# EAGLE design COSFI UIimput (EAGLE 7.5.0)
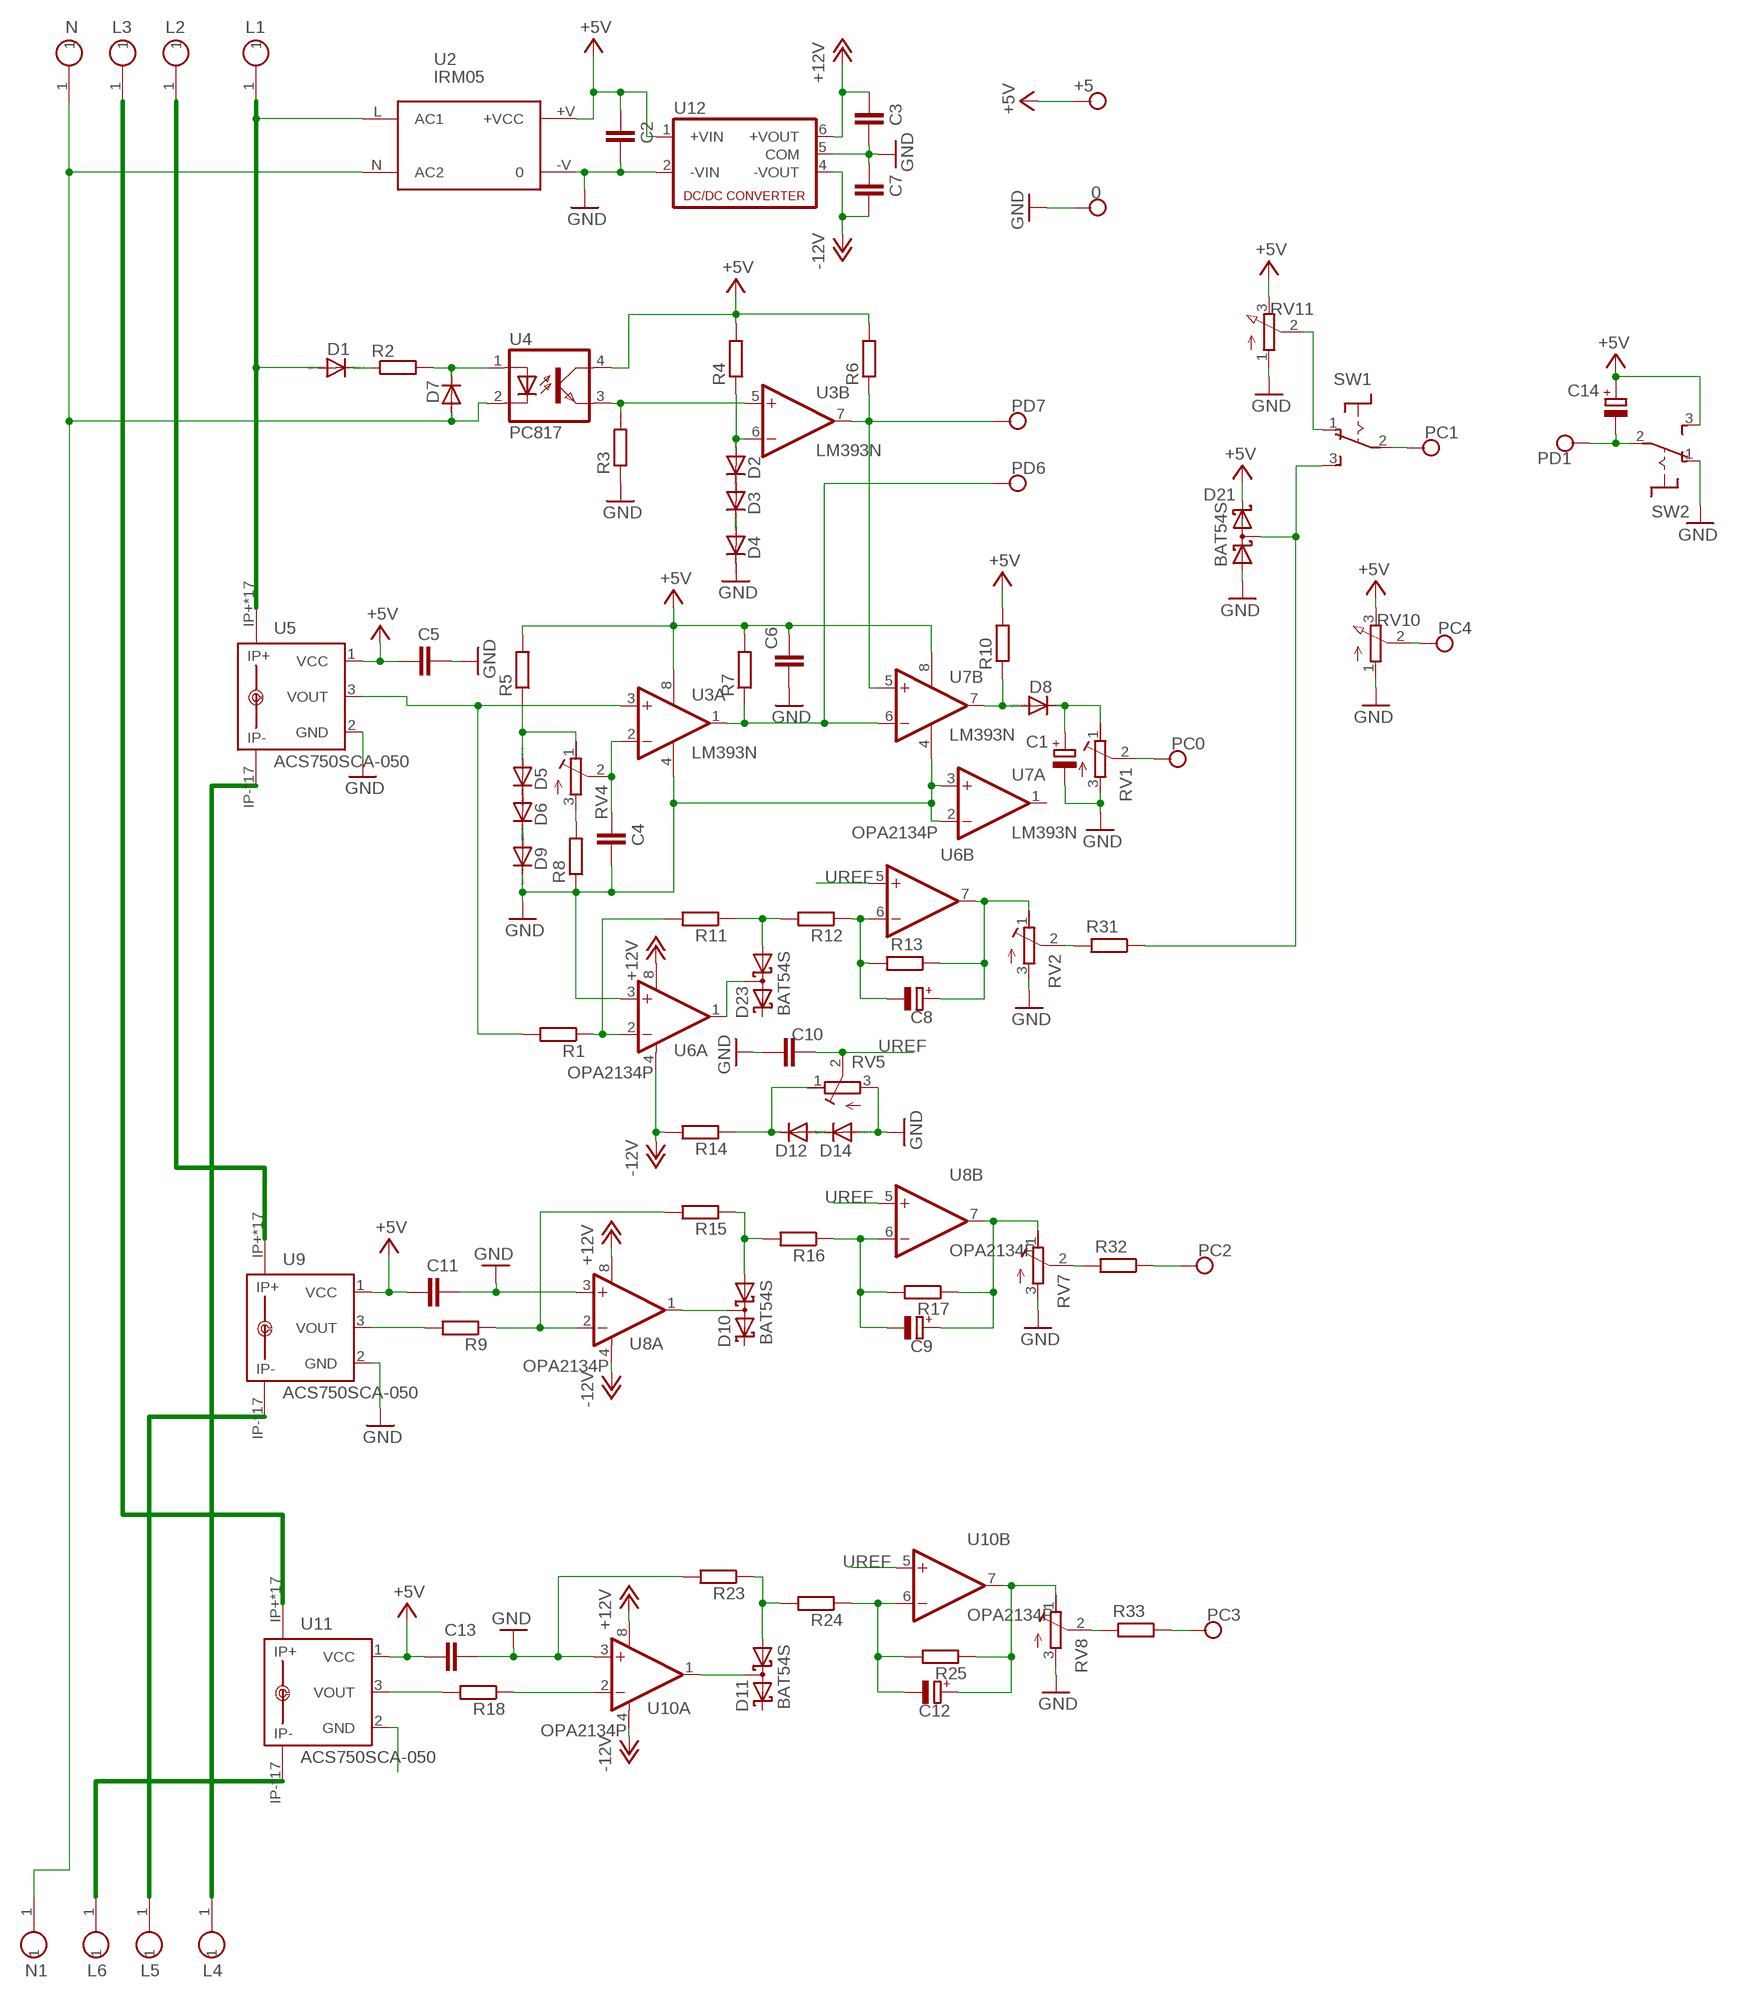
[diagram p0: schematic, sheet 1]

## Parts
0  CONNWIRE  [CONNWIRE]
+5  CONNWIRE  [CONNWIRE]
C1  CPOL-EUE2-5  [E2-5]
C2  C-EUC1206  [C1206]
C3  C-EUC1206  [C1206]
C4  C-EUC1206  [C1206]
C5  C-EUC1206  [C1206]
C6  C-EUC1206  [C1206]
C7  C-EUC1206  [C1206]
C8  CPOL-EUE2-5  [E2-5]
C9  CPOL-EUE2-5  [E2-5]
C10  C-EUC1206  [C1206]
C11  C-EUC1206  [C1206]
C12  CPOL-EUE2-5  [E2-5]
C13  C-EUC1206  [C1206]
C14  CPOL-EUE2-5  [E2-5]
D1  1N4004  [DO41-10]
D2  1N4148DO35-7  [DO35-7]
D3  1N4148DO35-7  [DO35-7]
D4  1N4148DO35-7  [DO35-7]
D5  1N4148DO35-7  [DO35-7]
D6  1N4148DO35-7  [DO35-7]
D7  1N4004  [DO41-10]
D8  1N4148DO35-7  [DO35-7]
D9  1N4148DO35-7  [DO35-7]
D10  BAT54S  [SOT23]
D11  BAT54S  [SOT23]
D12  1N4148DO35-7  [DO35-7]
D14  1N4148DO35-7  [DO35-7]
D21  BAT54S  [SOT23]
D23  BAT54S  [SOT23]
L1  CONNHOLE  [CONNHOLE4]
L2  CONNHOLE  [CONNHOLE4]
L3  CONNHOLE  [CONNHOLE4]
L4  CONNHOLE  [CONNHOLE4]
L5  CONNHOLE  [CONNHOLE4]
L6  CONNHOLE  [CONNHOLE4]
N  CONNHOLE  [CONNHOLE4]
N1  CONNHOLE  [CONNHOLE4]
PC0  CONNWIRE  [CONNWIRE]
PC1  CONNWIRE  [CONNWIRE]
PC2  CONNWIRE  [CONNWIRE]
PC3  CONNWIRE  [CONNWIRE]
PC4  CONNWIRE  [CONNWIRE]
PD1  CONNWIRE  [CONNWIRE]
PD6  CONNWIRE  [CONNWIRE]
PD7  CONNWIRE  [CONNWIRE]
R1  R-EU_0204/7  [0204/7]
R2  R-EU_0617/22  [0617/22]
R3  R-EU_0204/7  [0204/7]
R4  R-EU_0204/7  [0204/7]
R5  R-EU_0204/7  [0204/7]
R6  R-EU_0204/7  [0204/7]
R7  R-EU_0204/7  [0204/7]
R8  R-EU_0204/7  [0204/7]
R9  R-EU_0204/7  [0204/7]
R10  R-EU_0204/7  [0204/7]
R11  R-EU_0204/7  [0204/7]
R12  R-EU_0204/7  [0204/7]
R13  R-EU_0204/7  [0204/7]
R14  R-EU_0204/7  [0204/7]
R15  R-EU_0204/7  [0204/7]
R16  R-EU_0204/7  [0204/7]
R17  R-EU_0204/7  [0204/7]
R18  R-EU_0204/7  [0204/7]
R23  R-EU_0204/7  [0204/7]
R24  R-EU_0204/7  [0204/7]
R25  R-EU_0204/7  [0204/7]
R31  R-EU_0204/7  [0204/7]
R32  R-EU_0204/7  [0204/7]
R33  R-EU_0204/7  [0204/7]
RV1  R-TRIMM-3386-F  [R-TRIMM-3386F]
RV2  R-TRIMM-3386-F  [R-TRIMM-3386F]
RV4  R-TRIMM-3386-F  [R-TRIMM-3386F]
RV5  R-TRIMM-3386-F  [R-TRIMM-3386F]
RV7  R-TRIMM-3386-F  [R-TRIMM-3386F]
RV8  R-TRIMM-3386-F  [R-TRIMM-3386F]
RV10  PTV09A  PV09A  [PTV09]
RV11  PTV09A  PV09A  [PTV09]
SW1  8MS9P1  [8MS9]
SW2  8MS9P1  [8MS9]
U2  IRM05  [IRM05]
U3  LM393N  [DIL08]
U4  PC817  [DIL04]
U5  ACS750SCA-050  [ACS75050]
U6  OPA2134P  [DIL08]
U7  LM393N  [DIL08]
U8  OPA2134P  [DIL08]
U9  ACS750SCA-050  [ACS75050]
U10  OPA2134P  [DIL08]
U11  ACS750SCA-050  [ACS75050]
U12  NMA  [NMA]

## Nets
+5V: +5.P$1 C2.1 C5.2 C6.2 C11.2 C13.2 C14.+ D21.2(C2) R4.2 R5.2 R6.2 R7.2 R10.2 RV10.3(E) RV11.3(E) SW2.3(S) U2.+V(+VCC) U3.8(P:V+) U4.4(COL) U5.1(VCC) U7.8(P:V+) U9.1(VCC) U11.1(VCC) U12.1(+VIN)
+12V: C3.1 U6.8(A:V+) U8.8(A:V+) U10.8(A:V+) U12.6(+VOUT)
-12V: C7.2 R14.2 U6.4(A:V-) U8.4(A:V-) U10.4(A:V-) U12.4(-VOUT)
GND: 0.P$1 C1.- C2.2 C3.2 C4.2 C5.1 C6.1 C7.1 C10.1 C11.1 C13.1 D4.C D9.C D14.A D21.1(A1) R3.1 R8.1 R23.2 RV1.3(E) RV2.3(E) RV5.3(E) RV7.3(E) RV8.3(E) RV10.1(A) RV11.1(A) SW2.1(O) U2.-V U3.4(P:V-) U5.2(GND) U6.3(A:+IN) U7.2(A:-IN) U7.3(A:+IN) U7.4(P:V-) U8.3(A:+IN) U9.2(GND) U10.3(A:+IN) U11.2(GND) U12.2(-VIN) U12.5(COM)
N$1: D1.C R2.1
N$2: R1.1 R11.2 U6.2(A:-IN)
N$3: D7.C R2.2 U4.1(A)
N$4: D2.C D3.A
N$5: D7.A N1.1 N.1 U2.N(AC2) U4.2(C)
N$6: D1.A L1.1 U2.L(AC1) U5.IP+ U5.IP+@2(IP+) U5.IP+@3(IP+) U5.IP+@4(IP+) U5.IP+@5(IP+) U5.IP+@6(IP+) U5.IP+@7(IP+) U5.IP+@8(IP+) U5.IP+@9(IP+) U5.IP+@10(IP+) U5.IP+@11(IP+) U5.IP+@12(IP+) U5.IP+@13(IP+) U5.IP+@14(IP+) U5.IP+@15(IP+) U5.IP+@16(IP+) U5.IP+@17(IP+)
N$7: RV11.2(S) SW1.1(O)
N$8: D3.C D4.A
N$9: D12.A D14.C
N$10: D12.C R14.1 RV5.1(A)
N$11: R8.2 RV4.3(E)
N$12: D5.A R5.1 RV4.1(A)
N$13: R3.2 U3.5(B:+IN) U4.3(EMIT)
N$14: R1.2 U3.3(A:+IN) U5.3(VOUT)
N$15: D5.C D6.A
N$16: D2.A R4.1 U3.6(B:-IN)
N$17: D8.A R10.1 U7.7(B:OUT)
N$18: PD7.P$1 R6.1 U3.7(B:OUT) U7.5(B:+IN)
N$19: D6.C D9.A
N$20: PD6.P$1 R7.1 U3.1(A:OUT) U7.6(B:-IN)
N$21: C4.1 RV4.2(S) U3.2(A:-IN)
N$22: C1.+ D8.C RV1.1(A)
N$23: PC0.P$1 RV1.2(S)
N$24: D23.3(C1A2) U6.1(A:OUT)
N$25: PC1.P$1 SW1.2(P)
N$26: PC4.P$1 RV10.2(S)
N$27: D21.3(C1A2) R31.1 SW1.3(S)
N$28: C14.- PD1.P$1 SW2.2(P)
N$29: R9.1 R15.2 U8.2(A:-IN)
N$31: D23.1(A1) R11.1 R12.2
N$32: C8.- R12.1 R13.2 U6.6(B:-IN)
N$33: C8.+ R13.1 RV2.1(A) U6.7(B:OUT)
N$35: R31.2 RV2.2(S)
N$36: L2.1 U9.IP+ U9.IP+@2(IP+) U9.IP+@3(IP+) U9.IP+@4(IP+) U9.IP+@5(IP+) U9.IP+@6(IP+) U9.IP+@7(IP+) U9.IP+@8(IP+) U9.IP+@9(IP+) U9.IP+@10(IP+) U9.IP+@11(IP+) U9.IP+@12(IP+) U9.IP+@13(IP+) U9.IP+@14(IP+) U9.IP+@15(IP+) U9.IP+@16(IP+) U9.IP+@17(IP+)
N$37: D10.3(C1A2) U8.1(A:OUT)
N$39: R9.2 U9.3(VOUT)
N$40: D10.1(A1) R15.1 R16.2
N$41: C9.- R16.1 R17.2 U8.6(B:-IN)
N$42: C9.+ R17.1 RV7.1(A) U8.7(B:OUT)
N$43: PC2.P$1 R32.1
N$44: L3.1 U11.IP+ U11.IP+@2(IP+) U11.IP+@3(IP+) U11.IP+@4(IP+) U11.IP+@5(IP+) U11.IP+@6(IP+) U11.IP+@7(IP+) U11.IP+@8(IP+) U11.IP+@9(IP+) U11.IP+@10(IP+) U11.IP+@11(IP+) U11.IP+@12(IP+) U11.IP+@13(IP+) U11.IP+@14(IP+) U11.IP+@15(IP+) U11.IP+@16(IP+) U11.IP+@17(IP+)
N$45: R32.2 RV7.2(S)
N$46: R18.1 U10.2(A:-IN)
N$47: R18.2 U11.3(VOUT)
N$48: D11.3(C1A2) U10.1(A:OUT)
N$49: D11.1(A1) R23.1 R24.2
N$50: C12.- R24.1 R25.2 U10.6(B:-IN)
N$51: C12.+ R25.1 RV8.1(A) U10.7(B:OUT)
N$52: PC3.P$1 R33.1
N$53: R33.2 RV8.2(S)
N$54: L4.1 U5.IP- U5.IP-@2(IP-) U5.IP-@3(IP-) U5.IP-@4(IP-) U5.IP-@5(IP-) U5.IP-@6(IP-) U5.IP-@7(IP-) U5.IP-@8(IP-) U5.IP-@9(IP-) U5.IP-@10(IP-) U5.IP-@11(IP-) U5.IP-@12(IP-) U5.IP-@13(IP-) U5.IP-@14(IP-) U5.IP-@15(IP-) U5.IP-@16(IP-) U5.IP-@17(IP-)
N$55: L5.1 U9.IP- U9.IP-@2(IP-) U9.IP-@3(IP-) U9.IP-@4(IP-) U9.IP-@5(IP-) U9.IP-@6(IP-) U9.IP-@7(IP-) U9.IP-@8(IP-) U9.IP-@9(IP-) U9.IP-@10(IP-) U9.IP-@11(IP-) U9.IP-@12(IP-) U9.IP-@13(IP-) U9.IP-@14(IP-) U9.IP-@15(IP-) U9.IP-@16(IP-) U9.IP-@17(IP-)
N$57: L6.1 U11.IP- U11.IP-@2(IP-) U11.IP-@3(IP-) U11.IP-@4(IP-) U11.IP-@5(IP-) U11.IP-@6(IP-) U11.IP-@7(IP-) U11.IP-@8(IP-) U11.IP-@9(IP-) U11.IP-@10(IP-) U11.IP-@11(IP-) U11.IP-@12(IP-) U11.IP-@13(IP-) U11.IP-@14(IP-) U11.IP-@15(IP-) U11.IP-@16(IP-) U11.IP-@17(IP-)
UREF: C10.2 RV5.2(S) U6.5(B:+IN) U8.5(B:+IN) U10.5(B:+IN)
Unconnected: D10.2(C2) D11.2(C2) D23.2(C2) U7.1(A:OUT)

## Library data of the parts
0 +5 PC0 PC1-PC4 PD1 PD6 PD7 = connholes:CONNWIRE
C1 C8 C9 C12 C14 = rcl:CPOL-EU: POLARIZED CAPACITOR, European symbol
C2-C7 C10 C11 C13 = rcl:C-EU: CAPACITOR, European symbol
D1 D7 = diode:1N4004: DIODE
D2-D6 D8 D9 D12 D14 = diode:1N4148: DIODE
D10 D11 D21 D23 = diode:BAT54S: Schottky Diodes Pin connection corrected 2011-05-04 Source: Fairchild .. BAT54.pdf
L1-L6 N N1 = connholes:CONNHOLE
R1-R18 R23-R25 R31-R33 = rcl:R-EU_: RESISTOR, European symbol
RV1 RV2 RV4 RV5 RV7 RV8 = rcl:R-TRIMM-3386-F
RV10 RV11 = pot:PV09A
SW1 SW2 = switch:8MS9P1
U2 = acdc:IRM05: ACDC connector
U3 U7 = linear:LM393: COMPARATOR
U4 = optocoupler:PC817: SHARP OPTO COUPLER; MPN: PC817X4J000F; OC_FARNELL: 9707727; OC_NEWARK: 97K7059
U5 U9 U11 = allegro:ACS750*CA-050: Current Sensor display layer 49 Reference in BRD and place VIAs on circles Source: www.allegromicro.com/datafile/0750-050.pdf; MF: ALLEGRO MICROSYSTEMS, INC.; MPN: ACS750SCA-050; OC_FARNELL: 1457175; OC_NEWARK: 81H6588
U6 U8 U10 = burr-brown:OPA2134: Operational Amplifier; MF: TEXAS INSTRUMENTS; MPN: OPA2134PA; OC_FARNELL: 1097574; OC_NEWARK: 74K3897
U12 = dc-dc-converter:NMA: DC-DC CONVERTER; MF: C & D TECHNOLOGIES, INC; MPN: NMA0515SC; OC_FARNELL: 1021434; OC_NEWARK: 61K3064

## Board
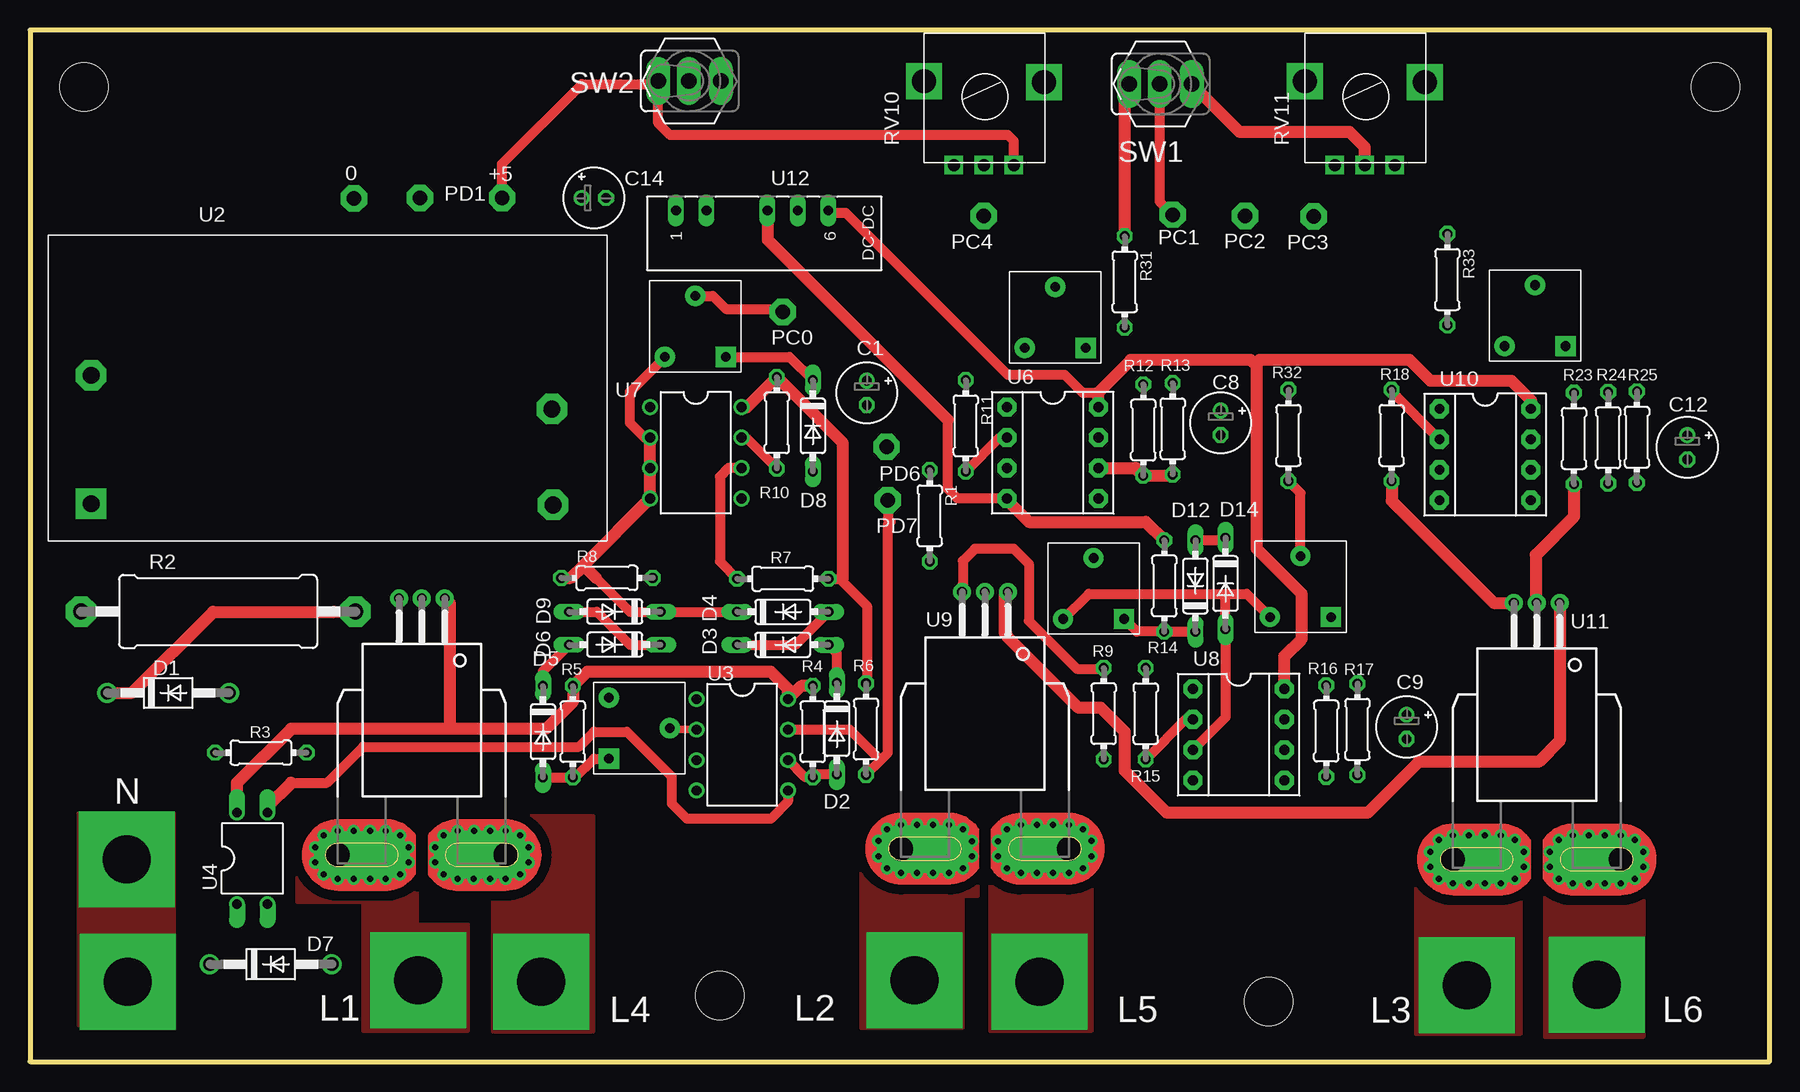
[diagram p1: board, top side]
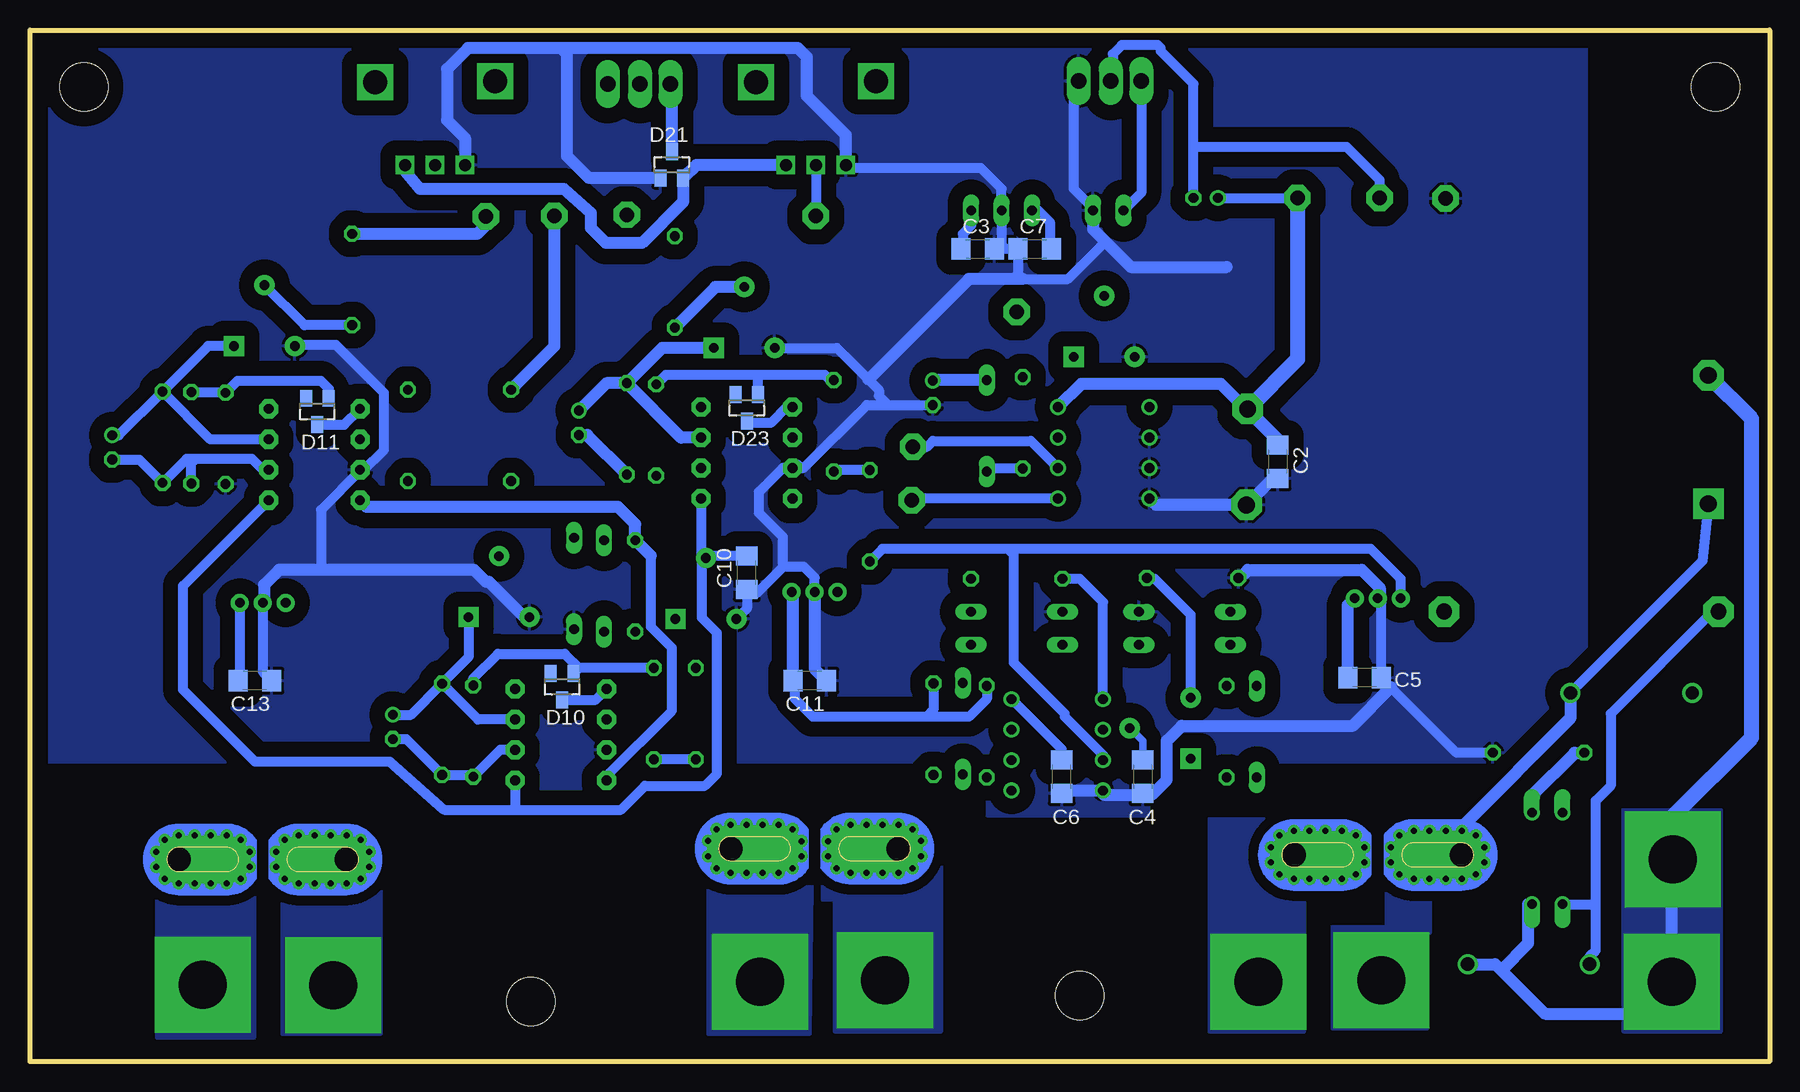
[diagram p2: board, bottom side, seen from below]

Size 145 x 86 mm. Coordinates in mm from the lower left corner, seen from the top.
Outline: 0,0 145,0 145,86 0,86 0,0
Copper layers (1*16): Top 0.035mm / dielectric 1.5mm / Bottom 0.035mm
Design rules "default": minimum track width 10mil, minimum drill 24mil, track to track 8mil, track to pad 8mil, pad to pad 8mil, via to via 8mil, smd to smd 8mil, copper to edge 40mil, drill to drill 8mil, minimum pad ring 10mil, minimum via ring 8mil, stop-mask expansion 4mil, vias tented up to drill 0mil, thermal gap 10mil
Holes 4 mm at 57.5,5.5 103.25,5 140.5,81.25 4.5,81.25
bRestrict: area 57.9,32.4 to 67.1,41.6

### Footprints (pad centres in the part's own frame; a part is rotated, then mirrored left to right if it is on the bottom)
CONNWIRE = drill 1.2 pad 2.184 octagon: P$1 0,0
E2-5 = drill 0.813 pad 1.27: + -1.016,0 | drill 0.813 pad 1.27 octagon: - 1.016,0
C1206 = smd 1.6 x 1.8: 1 -1.4,0; 2 1.4,0
DO41-10 = drill 1.118: A 5.08,0; C -5.08,0
DO35-7 = drill 0.813 long: A 3.81,0; C -3.81,0
SOT23 = smd 1 x 1.4: 1 -0.95,-1.1; 2 0.95,-1.1; 3 0,1.1
CONNHOLE4 = drill 4 pad 8 square: 1 0,0
0204/7 = drill 0.813 octagon: 1 -3.81,0; 2 3.81,0
0617/22 = drill 1.3 pad 2.54 octagon: 1 -11.43,0; 2 11.43,0
R-TRIMM-3386F = drill 0.8 pad 1.676 square: 1 0,0 | drill 0.8 pad 1.676: 2 5.08,2.54; 3 0,5.08
PTV09 = drill 1 square: 1 -2.5,0; 2 0,0; 3 2.5,0 | drill 2 square: P$4 -5,7; P$5 5,6.9
8MS9 = drill 1.295 pad 2 long: 1 -3,5.346 | drill 1.3 pad 2 long: 2 -3,2.654; 3 -3,0.114
IRM05 = drill 1.4 pad 2.54 octagon: +V 42,-14.5; -V 42.1,-22.5; N 3.6,-11.7 | drill 1.4 pad 2.54 square: L 3.6,-22.4
DIL08 = drill 0.813 pad 1.27: 1 -3.81,-3.81; 2 -1.27,-3.81; 3 1.27,-3.81; 4 3.81,-3.81; 5 3.81,3.81; 6 1.27,3.81; 7 -1.27,3.81; 8 -3.81,3.81
DIL04 = drill 0.813 offset: 1 -1.27,-3.81; 2 1.27,-3.81; 3 1.27,3.81; 4 -1.27,3.81
ACS75050 = drill 0.8 pad 1.5: 1 -1.91,-21.4; 2 0,-21.4; 3 1.91,-21.4 | drill 2 pad 4 offset: IP+ 7,0; IP- -7,0 | drill 0.5 pad 0.9: IP+@2 8.89,-0.635; IP+@3 8.89,0.635; IP+@4 8.175,1.625; IP+@5 7,2; IP+@6 5.675,2; IP+@7 4.325,2; IP+@8 3,2; IP+@9 1.825,1.625; IP+@10 1.1,0.625; IP+@11 1.1,-0.625; IP+@12 1.825,-1.625; IP+@13 3,-2; IP+@14 4.325,-2; IP+@15 5.675,-2; IP+@16 7,-2; IP+@17 8.175,-1.625; IP-@2 -8.89,-0.635; IP-@3 -8.89,0.635; IP-@4 -8.175,1.625; IP-@5 -7,2; IP-@6 -5.675,2; IP-@7 -4.325,2; IP-@8 -3,2; IP-@9 -1.825,1.625; IP-@10 -1.1,0.625; IP-@11 -1.1,-0.625; IP-@12 -1.825,-1.625; IP-@13 -3,-2; IP-@14 -4.35,-2; IP-@15 -5.675,-2; IP-@16 -7,-2; IP-@17 -8.175,-1.625
DIL08' = drill 0.813 pad 1.6 octagon: 1 -3.81,-3.81; 2 -1.27,-3.81; 3 1.27,-3.81; 4 3.81,-3.81; 5 3.81,3.81; 6 1.27,3.81; 7 -1.27,3.81; 8 -3.81,3.81
NMA = drill 0.813 long: 1 0,6.35; 2 0,3.81; 4 0,-1.27; 5 0,-3.81; 6 0,-6.35

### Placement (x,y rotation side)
0  27,71.95 0 top
+5  39.35,72 270 top
C1  69.75,55.75 270 top
C2  41,50 270 bottom
C3  66,67.75 0 bottom
C4  52.25,23.75 270 bottom
C5  33.75,32 180 bottom
C6  59,23.75 90 bottom
C7  61.25,67.75 0 bottom
C8  99.25,53.25 270 top
C9  114.75,27.9 270 top
C10  85.25,40.75 90 bottom
C11  80,31.75 180 bottom
C12  138.15,51.2 270 top
C13  126.25,31.75 180 bottom
C14  47,72 0 top
D1  11.52,30.73 0 top
D2  67.25,27.75 270 top
D3  62.75,34.75 0 top
D4  62.75,37.5 0 top
D5  42.75,27.5 270 top
D6  48.75,34.75 180 top
D7  20.07,8.11 0 top
D8  65.25,53 270 top
D9  48.75,37.5 180 top
D10  100.65,31.25 180 bottom
D11  121.05,54.2 180 bottom
D12  97.15,39.65 90 top
D14  99.65,39.85 270 top
D21  91.5,74.75 0 bottom
D23  85.25,54.5 180 bottom
L1  32.37,6.77 0 top
L2  73.73,6.77 0 top
L3  119.75,6.35 0 top
L4  42.6,6.65 0 top
L5  84.15,6.65 0 top
L6  130.6,6.4 0 top
N  8.05,16.85 0 top
N1  8.15,6.65 0 top
PC0  62.75,62.5 0 top
PC1  95.25,70.6 0 top
PC2  101.3,70.5 90 top
PC3  107,70.45 180 top
PC4  79.5,70.5 90 top
PD1  32.5,72 0 top
PD6  71.4,51.25 270 top
PD7  71.5,46.8 0 top
R1  75,45.5 270 top
R2  15.68,37.52 180 top
R3  19.25,25.75 180 top
R4  65.25,27.5 90 top
R5  45.25,27.5 90 top
R6  69.69,27.71 90 top
R7  62.75,40.25 0 top
R8  48.09,40.32 0 top
R9  89.5,29 90 top
R10  62.25,53.25 90 top
R11  78,53 270 top
R12  92.8,52.65 90 top
R13  95.25,52.75 270 top
R14  94.55,39.65 90 top
R15  93,29 270 top
R16  108.05,27.55 90 top
R17  110.65,27.7 270 top
R18  113.5,52.2 270 top
R23  128.7,51.95 270 top
R24  131.55,52 90 top
R25  133.95,52.05 270 top
R31  91.25,65 270 top
R32  104.9,52.2 270 top
R33  118.15,65.2 270 top
RV1  58,58.75 90 top
RV2  88,59.5 90 top
RV4  48.25,25.25 0 top
RV5  91.2,36.9 90 top
RV7  108.45,37.05 90 top
RV8  128,59.65 90 top
RV10  79.5,74.75 0 top
RV11  111.25,74.75 0 top
SW1  91.5,78.5 270 top
SW2  52.25,78.75 270 top
U2  1.5,68.9 0 top
U3  59.37,26.4 270 top
U4  18.53,16.93 0 top
U5  32.66,17.22 180 top
U6  OPA2134P  [DIL08']  85.25,50.75 270 top
U7  55.5,50.75 270 top
U8  OPA2134P  [DIL08']  100.75,27.25 270 top
U9  79.6,17.75 180 top
U10  OPA2134P  [DIL08']  121.3,50.6 270 top
U11  125.6,16.85 180 top
U12  60.2,70.95 90 top

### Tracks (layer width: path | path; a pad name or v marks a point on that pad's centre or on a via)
+5V
  Top 0.813: R6.2 69.75,31.58 69.75,38 67.5,40.25 R7.2 67.75,40.25 | RV10.3 82,76.75 81.5,77.25 53.36,77.25 52.36,78.25 52.36,80.89 51.75,81.5 | +5.P$1 39.35,74.85 46,81.5 51.75,81.5 | 51.75,81.5 52.11,81.5 SW2.3
  Top 1.016: U4.4 17.26,23.26 21.75,27.75 35,27.75 | R4.2 64.28,31.31 U3.8 63.18,31.07 61.75,32.5 46.44,32.5 R5.2 45.25,30 43,27.75 35,27.75 | 67.75,40.25 67.75,51.56 R10.2 59.75,54.56 U7.8 | 35,27.75 35,38.19 U5.1 | U11.1 127.51,26.76 125.75,25 115.75,25 111.5,20.75 94.75,20.75 91.25,24.25 91.25,27.5 89.25,29.5 87.4,29.5 81.4,35.5 81.4,35.6 81.25,35.75 81.25,38.89 U9.1
  Bottom 0.813: R4.2 65.25,30.25 66.75,28.75 70.25,28.75 | 70.25,28.75 79.75,28.75 81.25,30.25 81.25,31.6 C11.2 | R6.2 69.69,29.31 70.25,28.75 | C6.2 59,26.03 U3.8 | SW2.3 52.36,72.44 U12.1 53.98,71.08 | U11.1 127.51,31.89 C13.2 | C14.+ +5.P$1
  Bottom 1.016: C5.2 35.15,38.04 U5.1 | C11.2 81.4,39.04 U9.1 | U2.+V 41,51.9 C2.1 41,51.75 45.75,56.5 57.37,56.5 U7.8 | RV10.3 89.45,74.75 D21.2 | D21.2 90.55,72.2 | RV11.3 113.75,74.25 112.5,72.75 100.5,72.75 98.25,70.75 98.25,69.5 97,68.25 94,68.25 90.55,71.7 D21.2
  Bottom 1.27: +5.P$1 39.35,58.55 U2.+V
+12V
  Top 0.813: 89,55.75 87.75,55.75 86.25,57.25 81.5,57.25 68,70.75 66.75,70.75 U12.6
  Top 1.016: U8.8 104.56,33.81 106,35.25 106,39 102.25,42.75 102.25,58 102.12,58.12 | 102.12,58.12 101.75,58.5 91.75,58.5 89,55.75 89,54.62 U6.8 | U10.8 125.11,55.14 123.5,56.75 116.75,56.75 115,58.5 102.5,58.5 102.12,58.12
  Bottom 0.813: U12.6 66.55,69.7 67.25,69 67.25,67.9 C3.1
-12V
  Top 0.813: U6.4 77.31,46.94 76.5,47.75 76.5,53.5
  Top 1.016: 76.5,53.5 61.5,68.5 61.5,70.92 U12.4 | U6.4 81.44,46.81 83.25,45 93.01,45 R14.2
  Bottom 0.813: U12.4 60.95,70.95 60,70 60,67.9 C7.2 | U8.4 96.94,23.81 91.5,29.25 91.5,34.5 93.25,36.25 93.25,42.16
  Bottom 1.016: 93.25,42.16 R14.2 94.55,44.8 96,46.25 116.95,46.25 U10.4
GND
  Top 0.813: 47.18,40.32 50,37.5 D9.C D4.C | U7.2 51.23,52.02 50,53.25 50,55.83 RV1.3 | RV5.3 86.15,36.9 88.25,39 99.75,39 | 99.75,39 101.42,39 RV7.3 | 99.75,39 99.65,38.9 D14.A 99.65,28.69 U8.3
  Top 1.016: U7.2 U7.3 U7.4 46.12,41.38 | R8.1 45.07,40.32 46.12,41.38 | 47.18,40.32 46.12,41.38 | R23.2 128.7,45.45 125.5,42.25 125.5,38.35 U11.2
  Bottom 0.61: C4.2 55.32,22.35 U3.4 58.76,22.59 C6.1
  Bottom 0.813: R3.1 26.1,25.75 31.55,31.2 C5.1 32.35,38.31 U5.2 | 64,67.75 C7.1 62.65,65.65 62.25,65.25 58.5,65.25 55.38,68.38 | 64,67.75 C3.2 | 64,67.75 64.01,67.76 U12.5 64.01,72.76 65.75,74.5 76.75,74.5 RV10.1 | U9.2 79.6,40.35 80.5,41.25 82.25,41.25 | 82.25,41.25 84.5,39 84.9,39 C10.1 85.25,37.77 RV5.3 | 82.25,41.25 82.25,43.75 84.25,45.75 84.25,47.5 82.25,49.5 81.25,49.5 81,49.75 81.17,49.75 U6.3 80.52,49.48 75.25,54.75 73.5,54.75 | 73.5,54.75 69.77,54.75 C1.- | RV2.3 77.75,59.5 75.12,56.88 74.25,56 74.25,55.5 73.5,54.75 | U12.2 56.39,71.14 58,72.75 58,81.35 SW2.1 | 120.75,41 120.75,46 117.49,49.26 U10.3 117.17,49.33 115.5,51 115.5,55.75 119.5,59.75 122.82,59.75 RV8.3 | U11.2 125.6,32.5 C13.1
  Bottom 1.016: U9.2 79.6,32.75 C11.1 | R8.1 44.18,40.32 | 44.18,40.32 43.5,41 34,41 32.5,39.5 32.5,38.78 U5.2 | U7.4 51.15,46.4 U2.-V 41.4,48.6 C2.2 | 44.18,40.32 44.25,40.25 | U12.2 56.39,69.39 55.38,68.38 53.25,66.25 45.25,66.25 | 62.25,65.25 66.75,65.25 75.12,56.88 | RV7.3 103.8,37.05 106.75,40 107,40 108,41 120.75,41 124.25,41 125.5,39.75 125.5,38.35 U11.2 | 58.76,22.59 55.84,22.59 55.5,22.25 51.5,22.25 50.25,23.5 50.25,26.75 49,28 34.75,28 31.55,31.2 | RV10.1 77,77.25 80.25,80.5 80.25,83.75 81,84.5 100.75,84.5 | 100.75,84.5 108.5,84.5 110.25,82.75 110.25,78.5 108.75,77 RV11.1 | D21.1 98.4,73.65 100.25,75.5 100.25,84 100.75,84.5
  pour Bottom (isolate 1.27): 15.5,85 143.75,85 143.75,25 111.75,25 111.75,20.25 96.5,20.25 96.5,25 65.25,25 65.25,20.5 51.75,20.5 51.75,25 15.25,25 15.25,85.5
N$1
  Top 1.016: D1.C 8.48,30.73 15.25,37.5 25.34,37.5 R2.1
N$2
  Top 0.813: U6.2 80.83,52.02 R11.2
  Bottom 0.813: R1.1 77.88,49.31 R11.2
N$3
  Bottom 0.813: R2.2 4.73,37.52 13.25,29 13.25,23 14.5,21.75 14.5,13 | D7.C 14.99,8.76 14.5,9.25 14.5,13 | U4.1 14.62,13.12 14.5,13
N$4
  Top 0.813: D2.C 67.25,34.06 D3.A
N$5
  Bottom 0.813: U4.2 20.14,13.12
  Bottom 1.016: D7.A 22.86,8.11 22.38,7.62 | 22.38,7.62 18.75,4 10.8,4 N1.1 8.15,16.75 N.1 | 20.14,13.12 20.14,9.86 22.38,7.62
  Bottom 1.27: N.1 8.05,20.45 1.5,27 1.5,53.6 U2.N
  pour Top (isolate 0.813, no thermals): 4,20.75 12,20.75 12,3 4,3
  pour Bottom (isolate 0.813, no thermals): 4,21 12.25,21 12.25,2.5 4,2.5
N$6
  Bottom 0.813: U2.L 5.6,41.73 D1.A
  Bottom 1.016: D1.A 16.6,28.65 25.5,19.75 25.5,19.38 U5.IP+@16
  pour Bottom (isolate 0.813, no thermals): 22.5,20.25 32,20.25 32,19 32,11.25 36.5,11.25 36.5,2.75 28.5,2.75 28.5,10.75 28.25,10.75 28.25,13.75 22.25,13.75 22.25,20.25
  pour Top (isolate 0.813, no thermals): 22.25,20.25 32.25,20.25 32.25,11.5 36.5,11.5 36.5,2.5 27.75,2.5 27.75,13 27.75,13.25 22.25,13.25
N$7
  Top 1.016: RV11.2 111.25,76.25 110,77.5 100.85,77.5 SW1.1
N$8
  Top 0.813: D3.C 63.81,34.75 D4.A
N$9
  Top 0.813: D12.A 99.45,43.46 D14.C
N$10
  Top 0.813: RV5.1 92.26,35.84 R14.1 D12.C
N$11
  Bottom 0.813: RV4.3 48.25,37.25 51.25,40.25 51.83,40.25 R8.2
N$12
  Top 0.813: D5.A R5.1 45.44,23.69 47,25.25 RV4.1
N$13
  Top 0.813: 21.75,23.25 24.75,23.25 27.75,26.25 45.75,26.25 47,27.5 49.75,27.5 53.5,23.75 53.5,21.5 54.75,20.25 61.75,20.25 63.18,21.68 U3.5
  Top 1.016: U4.3 19.8,21.3 21.75,23.25
  Bottom 0.813: 19.8,22.2 U4.3
  Bottom 1.016: 19.8,22.2 16.25,25.75 R3.2
N$14
  Bottom 0.813: U5.3 30.75,40.25 33.25,42.75 63.5,42.75 | 63.5,42.75 73.94,42.75 R1.2 | U3.3 55.56,25.56 58.75,28.75 58.75,29 63,33.25 63,42.25 63.5,42.75
N$15
  Top 0.813: D5.C 42.75,32.56 D6.A
N$16
  Top 0.813: D2.A 65.5,23.94 R4.1 64.62,23.69 U3.6
N$17
  Top 0.813: U7.7 59.67,52.02 R10.1
  Bottom 0.813: R10.1 65,49.44 D8.A
N$18
  Top 0.813: R6.1 69.69,23.94 70.88,25.12 | 70.88,25.12 71.5,25.75 71.5,44.75 71.75,45 71.5,45.25 PD7.P$1 | U3.7 68.33,27.67 70.88,25.12
  Bottom 0.813: U7.5 71.36,46.94 PD7.P$1
N$19
  Top 0.813: D9.A 47.25,37.5 50,34.75 D6.C
N$20
  Top 0.813: U7.6 58.23,49.48 57.5,48.75 57.5,41.69 R7.1
  Bottom 0.813: U3.1 55.56,38.31 57.5,40.25 R7.1 | PD6.P$1 70.25,51.25 69.75,51.75 61.58,51.75 U7.6
N$21
  Top 0.61: U3.2 53.45,27.67 RV4.2
  Bottom 0.61: C4.1 52.25,26.71 RV4.2
N$22
  Top 0.813: RV1.1 63.31,58.75 D8.C
  Bottom 1.016: D8.C 69.71,56.81 C1.+
N$23
  Top 0.813: RV1.2 56.92,63.83 58,62.75 62.5,62.75 PC0.P$1
N$24
  Bottom 0.813: U6.1 81.94,54.56 83.25,53.25 85.1,53.25 D23.3
N$25
  Top 0.813: SW1.2 94.15,71.7 PC1.P$1
N$26
  Bottom 0.813: RV10.2 PC4.P$1
N$27
  Top 1.016: R31.1 91.25,81.14 SW1.3
  Bottom 1.016: D21.3 91.5,81.39 SW1.3
N$28
  Bottom 0.813: 55,81.65 SW2.2 54.75,81.9 54.75,84 54,84.75 51,84.75 50.75,84.5 50.75,84.25 48.02,81.52 48.02,76.25 | C14.- 48.02,76.25 | PD1.P$1 32.5,73.5 35.25,76.25 48.02,76.25
N$29
  Top 0.813: U8.2 96.33,28.52 R15.2
  Bottom 0.813: R9.1 R15.2
N$31
  Bottom 0.813: R11.1 78.31,56.81 78.75,57.25 84.25,57.25 | 84.25,57.25 92.01,57.25 R12.2 | D23.1 84.3,57.2 84.25,57.25
N$32
  Top 1.016: U6.6 92.16,49.48 R12.1 95.15,48.84 R13.2
  Bottom 1.016: C8.- 98.54,52.23 R13.2
N$33
  Bottom 1.016: U6.7 90.71,52.02 R13.1 | RV2.1 92.31,59.5 R13.1 | R13.1 96.96,56.56 C8.+
N$35
  Bottom 1.016: RV2.2 87.86,64.58 R31.2
N$36
  pour Top (isolate 0.813, no thermals): 69.5,20.75 79,20.75 79,15 79,13.75 77.75,13.75 77.75,2.75 69.25,2.75 69.25,20.75
  pour Bottom (isolate 0.813, no thermals): 69,21 79,21 79,13.5 78,13.5 78,2.5 69,2.5
N$37
  Bottom 0.813: D10.3 97.85,30.15 U8.1
N$39
  Top 0.813: U9.3 77.69,39.69 77.75,39.75 77.75,41.75 78.75,42.75 82,42.75 83.25,41.5 83.25,36.75 87.25,32.75 89.44,32.75 R9.2
N$40
  Bottom 0.813: R15.1 99.24,32.81 | 99.24,32.81 D10.1 | R16.2 108.05,31.95 106,34 100.43,34 99.24,32.81
N$41
  Bottom 0.813: C9.- 113.64,26.88 R17.2 108.2,23.89 R16.1 105.81,25.98 U8.6
N$42
  Bottom 0.813: U8.7 107.66,28.52 R17.1 | RV7.1 108.45,33.71 R17.1 | C9.+ 113.24,28.92 R17.1
N$43
  Bottom 1.016: PC2.P$1 101.3,59.61 R32.1
N$44
  pour Bottom (isolate 0.813, no thermals): 124,2.5 124,19.75 115.75,19.75 115.75,2.5 115.75,2.25 124,2.25
  pour Top (isolate 0.813, no thermals): 115.5,20 124.25,20 124.25,2.25 115.5,2.25
N$45
  Top 0.813: RV7.2 105.91,47.38 R32.2
N$46
  Top 0.813: R18.1 113.5,55.86 U10.2
N$47
  Top 1.016: R18.2 113.5,46.75 122,38.25 U11.3
N$48
  Bottom 0.813: D11.3 118.8,53.1 U10.1
N$49
  Bottom 0.813: D11.1 120.1,56.1 120.75,56.75 127.71,56.75 R23.1 131.5,55.76 R24.2
N$50
  Bottom 0.813: U10.6 125.58,49.33 126.5,50.25 131.25,50.25 | 131.25,50.25 131.94,50.25 R25.2 135.89,50.18 C12.- | R24.1 131.55,49.95 131.25,50.25
N$51
  Bottom 0.813: C12.+ 137.59,52.22 R25.1 | RV8.1 130.16,59.65 R25.1 | U10.7 129.96,51.87 R25.1
N$52
  Bottom 1.016: PC3.P$1 107,69.75 107.75,69 R33.1
N$53
  Bottom 0.813: R33.2 122.12,61.39 RV8.2
N$54
  pour Bottom (isolate 0.813, no thermals): 33.5,20.25 46.75,20.25 46.75,2.5 38.75,2.5 38.75,14 33.5,14 33.5,20
  pour Top (isolate 0.813, no thermals): 33.5,20.5 33.5,14 38.5,14 38.5,13.75 38.5,2.5 47,2.5 47,20.5
N$55
  pour Bottom (isolate 0.813, no thermals): 79.75,20.75 80,2.25 88.5,2.25 88.5,15 89.25,15 89.25,20.75
  pour Top (isolate 0.813, no thermals): 80,20.75 89.25,20.75 89.5,15 88.5,15 88.5,2.5 80,2.5
N$57
  pour Top (isolate 0.813, no thermals): 126.25,20 134.5,20 134.5,2 126.25,2
  pour Bottom (isolate 0.813, no thermals): 126.25,20 134.5,20 134.5,2 126.25,2
UREF
  Bottom 0.813: C10.2 88.49,42.15 RV5.2 | U6.5 89.06,42.38 RV5.2 | 104.75,21 110.5,21 115,25 126.25,25 132.25,31 132.25,39.65 U10.5 | 104.75,21 95.75,21 93.75,23 88.75,23 87.75,24 87.75,35.75 89,37 89,41.64 RV5.2 | U8.5 104.56,21.19 104.75,21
